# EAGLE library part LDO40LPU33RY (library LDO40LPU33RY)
LDO Voltage Regulators POWER MANAGEMENT Source: Datasheet
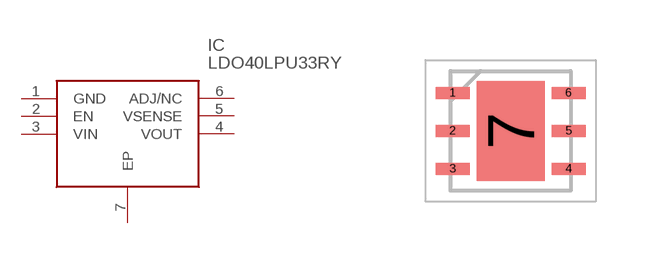
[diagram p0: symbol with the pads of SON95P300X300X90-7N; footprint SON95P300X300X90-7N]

Designator prefix IC

## LDO40LPU33RY (Description: LDO Voltage Regulators POWER MANAGEMENT; Height: 0.9mm; Manufacturer_Name: STMicroelectronics; Manufacturer_Part_Number: LDO40LPU33RY; Mouser_Part_Number: 511-LDO40LPU33RY; Mouser_Price-Stock: https://www.mouser.co.uk/ProductDetail/STMicroelectronics/LDO40LPU33RY?qs=qSfuJ%252Bfl%2Fd5qazWclm%2Ffpg%3D%3D)  [SON95P300X300X90-7N]
1  GND
2  EN
3  VIN
4  VOUT
5  VSENSE
6  ADJ/NC
7  EP

## Footprint SON95P300X300X90-7N (pad centres in mm)
LDO40LPU33RY_
smd 0.85 x 0.3: 1 -1.45,0.95; 2 -1.45,0; 3 -1.45,-0.95; 4 1.45,-0.95; 5 1.45,0; 6 1.45,0.95
smd 1.7 x 2.5: 7 0,0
